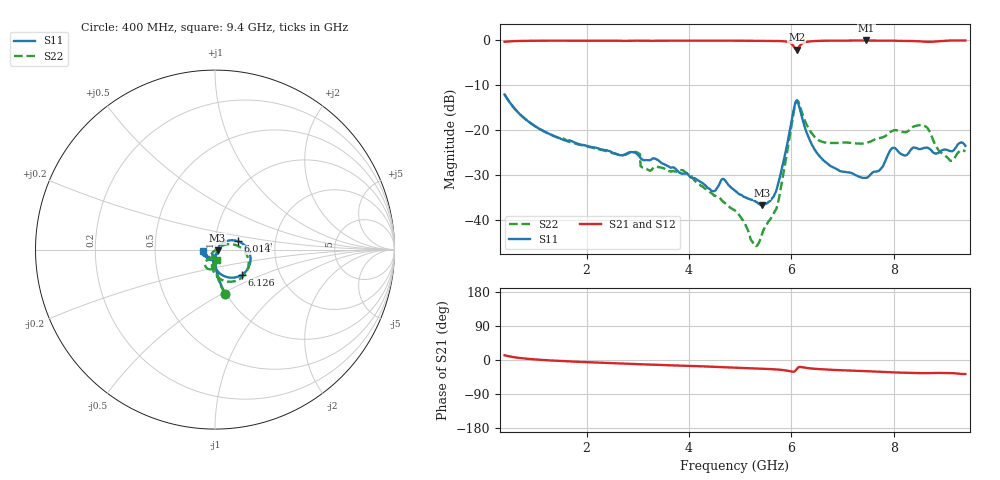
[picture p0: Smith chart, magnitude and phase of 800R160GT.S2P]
!  American Technical Ceramics  Date:  6/19/09
!  One Norden Lane
!  Huntington Station,  NY.  11746-2102
!  Tel:  (631) 622-4700  Fax:  (631) 622-4748
!  Part Number  800R160GT
!  Description: Ultra-low ESR, NPO  Mounting Orientation: Vertical
!  Application: High RF power Filters, Combiners, Matching networks,
!  Antenna, DC block, Bypass and Couplers
# GHZ S DB R 50
! Freq  |S11|  S11 Ph  |S21|  S21 Ph  |S12|  S12 Ph  |S22|  S22 Ph
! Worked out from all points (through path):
!   801 points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, 400 MHz to 9.4 GHz, reference 50 ohm
!   highest |S21| = 0.00 dB at 7.465 GHz (marker M1); lowest = -2.0 dB at 6.104 GHz (marker M2)
!   group delay of S21, straight-line fit = 12.7 ps
!   lowest |S11| = -36.6 dB at 5.429 GHz (marker M3), VSWR 1.03, Z = 51.4 - j0.467 ohm
!   |S11| at or under -10 dB: start of sweep to end of sweep
!   |S22| runs from -45.8 to -12.0 dB; largest |S21 - S12| = 0.0016
!   S11 on the Smith chart (normalised r, x): 400 MHz: 0.99, -0.51; 6.014 GHz: 1.28, +0.12; 6.126 GHz: 1.29, -0.38; 9.4 GHz: 0.88, -0.02
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0.4  -12.00 -77.1  -0.29 12.5  -0.29 12.6  -12.01 -77.4
0.996  -19.06 -87.1  -0.07 1.5  -0.07 1.5  -19.09 -89.3
1.908  -23.20 -89.2  -0.05 -5.2  -0.05 -5.2  -23.29 -99.2
2.965  -25.07 -85.6  -0.05 -10.7  -0.05 -10.7  -24.80 -114.5
3.1  -26.55 -86.5  -0.04 -11.5  -0.04 -11.5  -28.33 -108.7
3.404  -26.66 -87.9  -0.05 -12.8  -0.05 -12.8  -28.17 -106.2
3.899  -29.63 -81.0  -0.08 -15.2  -0.08 -15.2  -28.99 -119.9
4.461  -33.53 -61.9  -0.04 -17.8  -0.04 -17.8  -34.20 -130.8
4.9  -33.41 -57.8  -0.06 -20.1  -0.06 -20.2  -37.83 -124.7
5.271  -35.60 -35.6  -0.09 -22.1  -0.08 -22.1  -45.27 -88.3
5.429  -36.63 -17.9  -0.10 -23.0  -0.10 -23.0  -42.95 -40.5
5.733  -32.34 33.6  -0.13 -25.1  -0.13 -25.1  -36.42 11.1
6.014  -17.41 20.4  -0.85 -30.7  -0.85 -30.8  -18.10 10.4
6.104  -13.46 -28.2  -2.05 -24.1  -2.05 -24.1  -13.32 -36.4
6.126  -13.73 -43.1  -1.83 -20.6  -1.83 -20.6  -13.39 -50.9
6.408  -23.30 -99.4  -0.17 -22.6  -0.17 -22.6  -20.78 -100.8
6.779  -27.97 -108.3  -0.06 -25.8  -0.05 -25.9  -22.79 -98.6
7.465  -30.53 -111.3  0.00 -29.4  -0.01 -29.4  -22.78 -93.8
7.904  -25.04 -105.4  -0.01 -32.3  -0.01 -32.3  -20.65 -89.1
8.568  -24.01 -141.2  -0.23 -34.8  -0.23 -34.9  -18.88 -111.0
9.096  -24.58 -149.4  0.00 -34.5  0.00 -34.5  -26.64 -98.2
9.4  -23.44 -171.5  -0.01 -37.1  -0.01 -37.1  -24.67 -78.3
